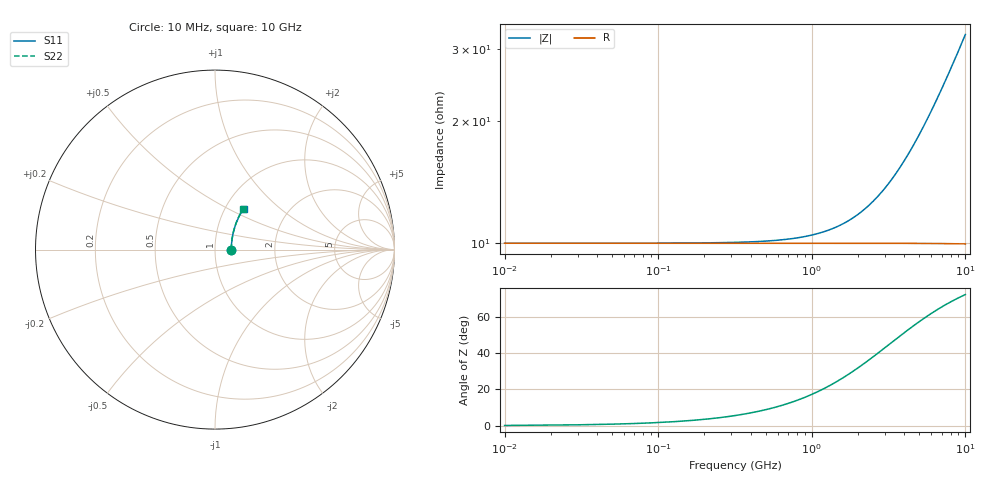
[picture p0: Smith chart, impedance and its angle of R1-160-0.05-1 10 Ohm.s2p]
!version-1
!date-03.2021
# MHz S RI R 50
!Freq ReS11 ImS11 ReS21 ImS21 ReS12 ImS12 ReS22 ImS22
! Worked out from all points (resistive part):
!   501 points, 10 MHz to 10 GHz, reference 50 ohm
!   read as one part in series: R = 10 ohm at 50 MHz
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10  0.0909 0.000247  0.9091 -0.000267  0.9091 -0.000267  0.0909 0.000247
190  0.0909 0.00468  0.9091 -0.00506  0.9091 -0.00506  0.0909 0.0047
390  0.091 0.00961  0.909 -0.0104  0.909 -0.0104  0.091 0.00965
590  0.0912 0.0145  0.9088 -0.0157  0.9088 -0.0157  0.0912 0.0146
790  0.0914 0.0195  0.9086 -0.021  0.9086 -0.021  0.0914 0.0195
990  0.0916 0.0244  0.9084 -0.0264  0.9084 -0.0264  0.0916 0.0245
1210  0.092 0.0298  0.908 -0.0322  0.908 -0.0322  0.092 0.0299
1450  0.0924 0.0357  0.9076 -0.0386  0.9076 -0.0386  0.0924 0.0358
1690  0.093 0.0416  0.907 -0.0449  0.907 -0.0449  0.093 0.0417
1990  0.0938 0.0489  0.9062 -0.0529  0.9062 -0.0529  0.0937 0.0491
2350  0.0949 0.0577  0.9051 -0.0624  0.9051 -0.0624  0.0949 0.0579
3350  0.0991 0.0818  0.901 -0.0885  0.901 -0.0885  0.0989 0.0821
4250  0.104 0.1032  0.8961 -0.1117  0.8961 -0.1117  0.1037 0.1036
5010  0.109 0.121  0.8912 -0.131  0.8912 -0.131  0.1086 0.1215
5830  0.1152 0.1397  0.885 -0.1514  0.885 -0.1514  0.1147 0.1404
6250  0.1187 0.1492  0.8815 -0.1617  0.8815 -0.1617  0.1181 0.1499
6670  0.1225 0.1585  0.8778 -0.1719  0.8778 -0.1719  0.1218 0.1593
7490  0.1303 0.1763  0.87 -0.1914  0.87 -0.1914  0.1295 0.1772
8350  0.1394 0.1944  0.861 -0.2113  0.861 -0.2113  0.1383 0.1955
9210  0.1492 0.2119  0.8512 -0.2305  0.8512 -0.2305  0.1479 0.2131
9710  0.1553 0.2217  0.8452 -0.2414  0.8452 -0.2414  0.1539 0.223
10000  0.1589 0.2273  0.8417 -0.2476  0.8417 -0.2476  0.1574 0.2287
